TYPE Alm_AlarmType :
STRUCT
      (*InPut*)
	EventId:					INT;
    EventMessage:			WSTRING;
    EventTime:                                 DT;
	EventActive:				BOOL;
	QuitRequired:				BOOL;
	QuitEvent:				BOOL;
	EventClass:				Alm_EventClass;
	AlarmMsg:				Alm_AlmMsg;
	AlarmlampOn:			BOOL;(*报警灯*)
	AutoRunOff:				BOOL;(*退出自动循环*)

	(* event actions OutPut	*)
	AlarmAction1:				BOOL;
	AlarmAction2:				BOOL;
	AlarmAction3:				BOOL;
	AlarmAction4:				BOOL;
	AlarmAction5:				BOOL;
	AlarmAction6:				BOOL;
	AlarmAction7:				BOOL;
	AlarmAction8:				BOOL;

       (*OutPut*)
	EventAlive:					BOOL;
    ShowlampOn:           		BOOL;
	InUse:                		BOOL;
END_STRUCT
END_TYPE;
